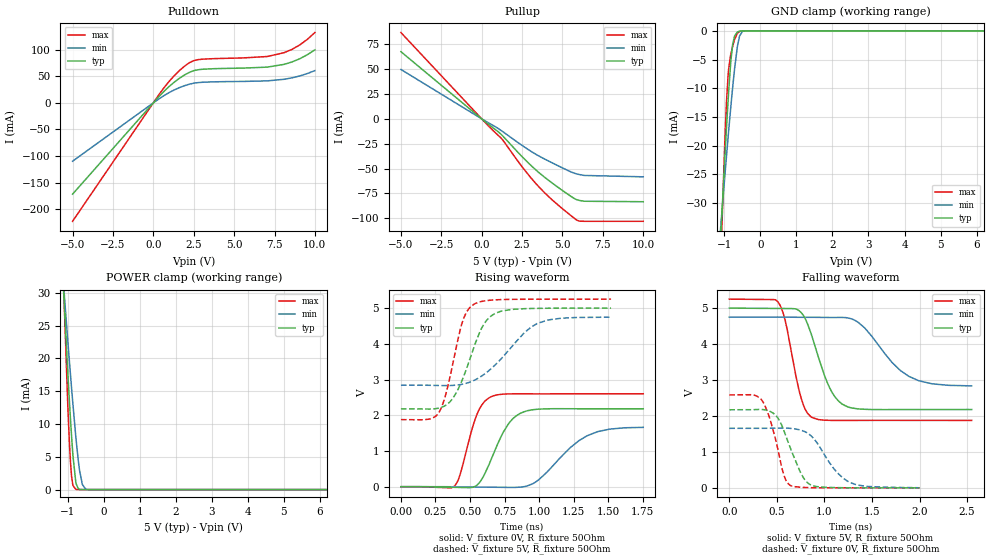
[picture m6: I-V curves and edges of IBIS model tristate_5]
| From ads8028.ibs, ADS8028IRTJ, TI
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|   tristate_5 Model
[Model]   tristate_5
Model_type   3-state
Polarity   Non-Inverting
Vmeas = 2.5
Vref = 0
Cref = 15pF
Rref = 150
|   typ   min   max
|   (nom PVT)   (fast PVT)   (slow PVT)
C_comp   1.153e-12   9.341e-13   1.384e-12
| Where nom  PVT is Nominal Process, 5V, 27C
|   Fast PVT is Strong Process,  5.25V, -40C
|   Slow PVT is Weak Process,   4.75V, 125C
[Voltage Range]   5   4.75   5.25
|Junction Temperature
[Temperature Range]   27   125   -40
[Pullup Reference]   5   4.75   5.25
[Pulldown Reference]   0   0   0
[Power Clamp Reference]   5   4.75   5.25
[GND Clamp Reference]   0   0   0
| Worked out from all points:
|   slope of the pulldown table from 0 to 0.75 V, typ, clamps not added: 30.9 ohm
|   slope of the pullup table from 0 to 0.75 V, typ, clamps not added: 77.8 ohm
|   GND clamp passes 1 mA (typ) near -0.72 V on its own axis
|   POWER clamp passes 1 mA (typ) near -0.77 V on its own axis
|   falling waveform, V_fixture 5V, R_fixture 50Ohm: 20-80 % time 223ps typ, 374ps min, 155ps max; typ from 5 V to 2.18 V
|   rising waveform, V_fixture 0V, R_fixture 50Ohm: 20-80 % time 160ps typ, 270ps min, 115ps max; typ from 0 V to 2.18 V
|   rising waveform, V_fixture 5V, R_fixture 50Ohm: 20-80 % time 168ps typ, 283ps min, 120ps max; typ from 2.18 V to 5 V
|   falling waveform, V_fixture 0V, R_fixture 50Ohm: 20-80 % time 196ps typ, 269ps min, 149ps max; typ from 2.17 V to 0 V
[Pulldown]
|   Voltage   I(typ)   I(min)   I(max)
-5V       -171.3mA   -109.5mA   -222.3mA
400mV     13.54mA    8.57mA     17.74mA
1.3V      38.97mA    24.32mA    51.1mA
1.972V    53.02mA    32.64mA    69.74mA
2.265V    57.67mA    35.27mA    75.84mA
2.75V     62.06mA    37.93mA    81mA
7.04V     67.06mA    41.24mA    86.95mA
8.09V     72.24mA    44.24mA    94.13mA
8.592V    76.88mA    46.98mA    100.5mA
9.065V    82.83mA    50.53mA    108.8mA
9.532V    90.36mA    55.04mA    119.2mA
10V       99.48mA    60.53mA    131.9mA
[GND Clamp]
|   Voltage   I(typ)   I(min)   I(max)
-5V       -577.7mA   -377.4mA   -895.1mA
-1.129V   -39.12mA   -36.21mA   -45.24mA
-994.2mV  -22.83mA   -25.76mA   -20.36mA
-941.7mV  -16.87mA   -21.81mA   -12.41mA
-885mV    -10.91mA   -17.67mA   -6.807mA
-820mV    -5.226mA   -13.12mA   -4.044mA
-770mV    -2.344mA   -9.817mA   -2.687mA
-720mV    -954.7uA   -6.764mA   -1.58mA
-639.5mV  -214.7uA   -2.736mA   -445.6uA
-577.7mV  -55.26uA   -887.2uA   -112.9uA
-359.3mV  -144.8nA   -2.375uA   -135.3nA
10V       0A         0A         0A
[Pullup]
|   Voltage   I(typ)   I(min)   I(max)
-5V       67.61mA    49.72mA    86.88mA
163.3mV   -2.184mA   -1.589mA   -2.836mA
1.258V    -16.53mA   -12.34mA   -20.46mA
2.55V     -38.92mA   -27.34mA   -49.32mA
3.602V    -54.94mA   -37.96mA   -69.54mA
4.357V    -64.58mA   -44.26mA   -81.52mA
5.78V     -80.68mA   -54.96mA   -100.7mA
6.02V     -82.03mA   -55.98mA   -102.9mA
6.343V    -82.94mA   -56.98mA   -103.1mA
10V       -83.44mA   -58.36mA   -103.1mA
[POWER Clamp]
|   Voltage   I(typ)   I(min)   I(max)
-5V       422mA      299.4mA    614.5mA
-1.18V    37.56mA    36.02mA    41.53mA
-994.2mV  17.63mA    22.53mA    12.56mA
-950mV    13.35mA    19.46mA    7.015mA
-920.7mV  10.68mA    17.46mA    4.11mA
-889.2mV  7.984mA    15.34mA    1.939mA
-857.8mV  5.547mA    13.27mA    778.4uA
-775mV    1.187mA    8.148mA    53.11uA
-672.7mV  41.33uA    3.036mA    1.655uA
-592mV    2.175uA    785.2uA    109.1nA
-463.7mV  24.96nA    27.57uA    0A
10V       0A         0A         0A
[Ramp]
R_load = 50
|   typ   min   max
dV/dt_r   1.30668/1.59436e-10   0.995337/2.65792e-10   1.55667/1.14478e-10
dV/dt_f   1.69253/2.21949e-10   1.14578/3.67278e-10   2.02372/1.54611e-10
[Falling Waveform]
V_fixture = 5V
V_fixture_min = 4.75V
V_fixture_max = 5.25V
R_fixture = 50Ohm
|   Time   V(typ)   V(min)   V(max)
0s        5V         4.75V      5.25V
512ps     4.991V     4.751V     5.169V
588ps     4.989V     4.749V     4.652V
756ps     4.873V     4.744V     2.491V
876ps     4.158V     4.744V     1.951V
1.056ns   2.777V     4.739V     1.878V
1.228ns   2.274V     4.735V     1.876V
1.422ns   2.186V     4.453V     1.878V
1.89ns    2.178V     3.099V     1.878V
2.548ns   2.179V     2.837V     1.877V
[Rising Waveform]
V_fixture = 0V
V_fixture_min = 0V
V_fixture_max = 0V
R_fixture = 50Ohm
|   Time   V(typ)   V(min)   V(max)
0s        2.398nV    4.467nV    2.071nV
388ps     -17.24mV   -2.522mV   17.22mV
428ps     -20.98mV   -4.316mV   339mV
554ps     56.9mV     -10.95mV   2.06V
656ps     792.4mV    -14.53mV   2.524V
774ps     1.735V     -19.42mV   2.597V
900ps     2.109V     7.708mV    2.599V
1ns       2.171V     203.5mV    2.599V
1.346ns   2.181V     1.423V     2.6V
1.754ns   2.181V     1.661V     2.6V
[Rising Waveform]
V_fixture = 5V
V_fixture_min = 4.75V
V_fixture_max = 5.25V
R_fixture = 50Ohm
|   Time   V(typ)   V(min)   V(max)
0s        2.179V     2.84V      1.877V
204ps     2.173V     2.839V     1.891V
278ps     2.203V     2.832V     2.1V
334ps     2.304V     2.83V      2.725V
440ps     2.954V     2.865V     4.55V
528ps     3.898V     2.974V     5.106V
612ps     4.614V     3.173V     5.205V
722ps     4.909V     3.565V     5.236V
990ps     4.992V     4.574V     5.248V
1.521ns   5V         4.75V      5.25V
[Falling Waveform]
V_fixture = 0V
V_fixture_min = 0V
V_fixture_max = 0V
R_fixture = 50Ohm
|   Time   V(typ)   V(min)   V(max)
0s        2.172V     1.657V     2.586V
348ps     2.178V     1.657V     2.415V
508ps     1.954V     1.663V     1.107V
584ps     1.519V     1.663V     279.3mV
642ps     1.11V      1.655V     66.81mV
778ps     287.4mV    1.582V     12.87mV
864ps     70.86mV    1.437V     4.814mV
1.132ns   6.599mV    431mV      901.2uV
1.268ns   2.126mV    150.5mV    720.3uV
2ns       413.7uV    3.036mV    214.5uV
